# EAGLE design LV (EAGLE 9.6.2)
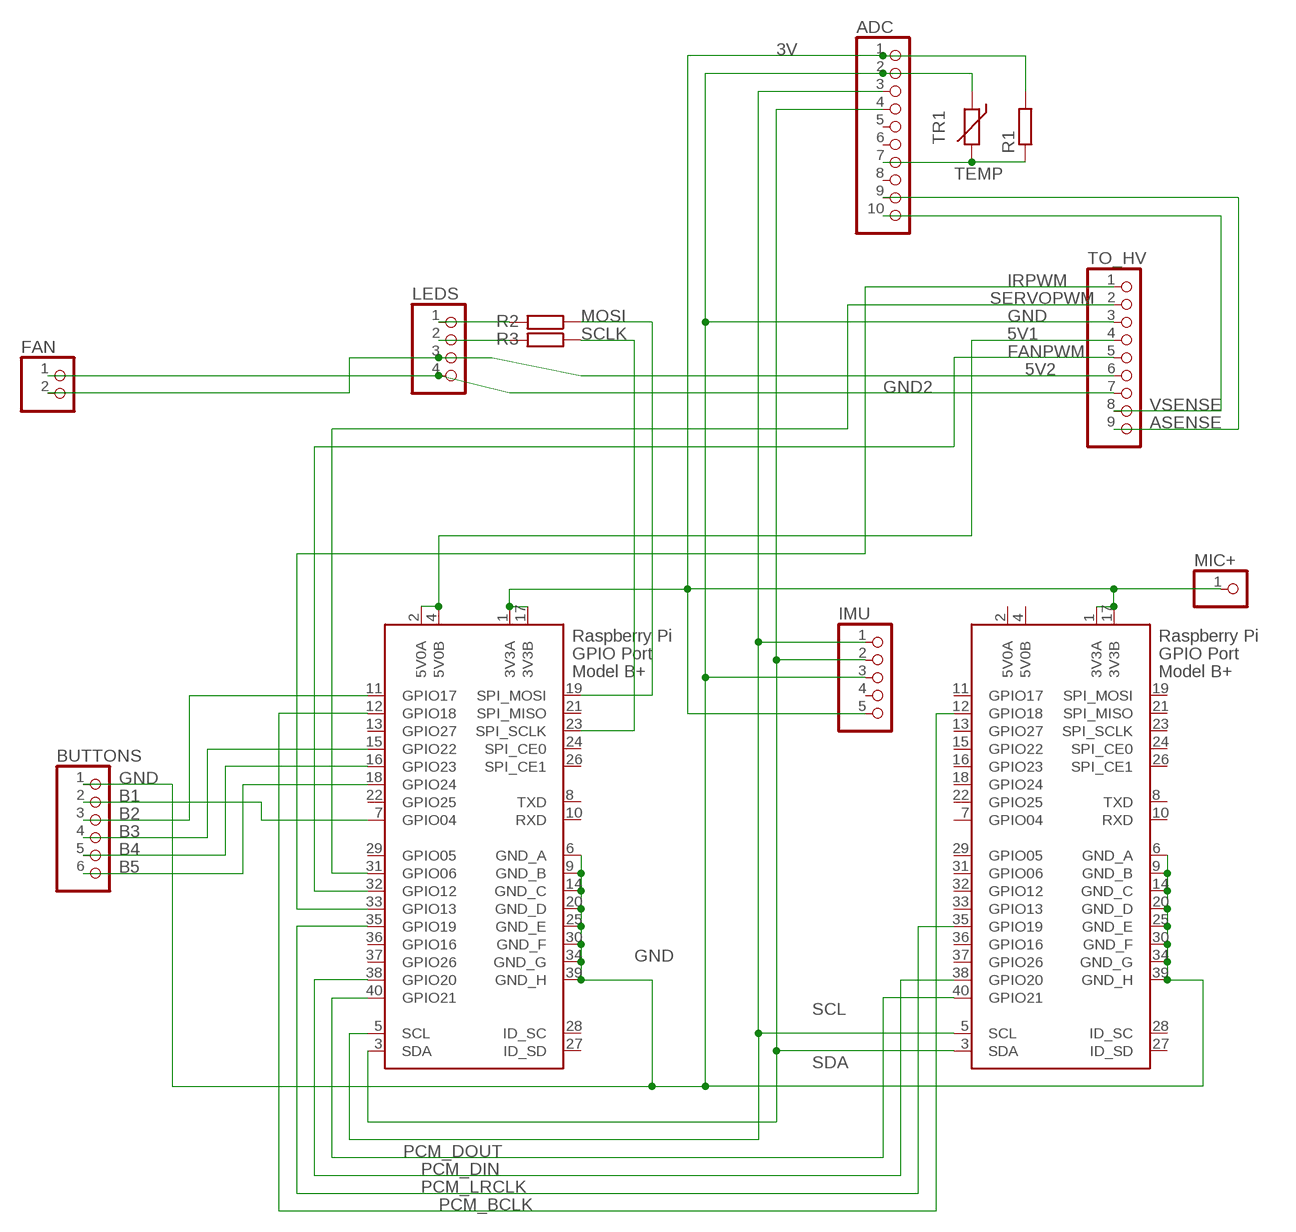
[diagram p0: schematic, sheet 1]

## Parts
ADC  PINHD-1X10  [1X10]
BUTTONS  PINHD-1X6  [1X06]
FAN  PINHD-1X2  [1X02]
IMU  PINHD-1X5  [1X05]
LEDS  PINHD-1X4  [1X04]
MIC+  PINHD-1X1  [1X01]
R1  R-EU_0204/7  [0204/7]
R2  R-EU_0204/7  [0204/7]
R3  R-EU_0204/7  [0204/7]
TO_HV  PINHD-1X9  [1X09]
TR1  THERMISTOR_R-2,5  [RS-2,5]
X1  RASPI_BOARD_B+#_E4P  [RASPI_BOARD_B+_EDGES_4DRILL_PAD]
X2  RASPI_BOARD_B+#F  [FE-PI]

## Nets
3V [PWR]: ADC.1 IMU.5 MIC+.1 R1.2 X1.1(3V3A) X1.17(3V3B) X2.1(3V3A) X2.17(3V3B)
5V1 [PWR]: TO_HV.4 X1.2(5V0A) X1.4(5V0B)
5V2 [PWR]: FAN.2 LEDS.3 TO_HV.6
ASENSE: ADC.9 TO_HV.9
B1: BUTTONS.2 X1.7(GPIO04)
B2: BUTTONS.3 X1.11(GPIO17)
B3: BUTTONS.4 X1.15(GPIO22)
B4: BUTTONS.5 X1.16(GPIO23)
B5: BUTTONS.6 X1.18(GPIO24)
FANPWM: TO_HV.5 X1.32(GPIO12)
GND [PWR]: ADC.2 BUTTONS.1 IMU.3 TO_HV.3 TR1.1 X1.6(GND_A) X1.9(GND_B) X1.14(GND_C) X1.20(GND_D) X1.25(GND_E) X1.30(GND_F) X1.34(GND_G) X1.39(GND_H) X2.6(GND_A) X2.9(GND_B) X2.14(GND_C) X2.20(GND_D) X2.25(GND_E) X2.30(GND_F) X2.34(GND_G) X2.39(GND_H)
GND2 [PWR]: FAN.1 LEDS.4 TO_HV.7
IRPWM: TO_HV.1 X1.33(GPIO13)
MOSI: R2.1 X1.19(SPI_MOSI)
N$6: LEDS.2 R3.2
N$7: LEDS.1 R2.2
PCM_BCLK: X1.12(GPIO18) X2.12(GPIO18)
PCM_DIN: X1.38(GPIO20) X2.38(GPIO20)
PCM_DOUT: X1.40(GPIO21) X2.40(GPIO21)
PCM_LRCLK: X1.35(GPIO19) X2.35(GPIO19)
SCL: ADC.3 IMU.1 X1.5(SCL) X2.5(SCL)
SCLK: R3.1 X1.23(SPI_SCLK)
SDA: ADC.4 IMU.2 X1.3(SDA) X2.3(SDA)
SERVOPWM: TO_HV.2 X1.31(GPIO06)
TEMP: ADC.7 R1.1 TR1.2
VSENSE: ADC.10 TO_HV.8
Unconnected: ADC.5 ADC.6 ADC.8 IMU.4 X1.8(TXD) X1.10(RXD) X1.13(GPIO27) X1.21(SPI_MISO) X1.22(GPIO25) X1.24(SPI_CE0) X1.26(SPI_CE1) X1.27(ID_SD) X1.28(ID_SC) X1.29(GPIO05) X1.36(GPIO16) X1.37(GPIO26) X2.7(GPIO04) X2.8(TXD) X2.10(RXD) X2.11(GPIO17) X2.13(GPIO27) X2.15(GPIO22) X2.16(GPIO23) X2.18(GPIO24) X2.19(SPI_MOSI) X2.21(SPI_MISO) X2.22(GPIO25) X2.23(SPI_SCLK) X2.24(SPI_CE0) X2.26(SPI_CE1) X2.27(ID_SD) X2.28(ID_SC) X2.29(GPIO05) X2.31(GPIO06) X2.32(GPIO12) X2.33(GPIO13) X2.36(GPIO16) X2.37(GPIO26)

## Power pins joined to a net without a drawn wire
5V0A: X2.2(5V0A)
5V0B: X2.4(5V0B)

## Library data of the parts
ADC = pinhead:PINHD-1X10: PIN HEADER
BUTTONS = pinhead:PINHD-1X6: PIN HEADER
FAN = pinhead:PINHD-1X2: PIN HEADER
IMU = pinhead:PINHD-1X5: PIN HEADER
LEDS = pinhead:PINHD-1X4: PIN HEADER
MIC+ = pinhead:PINHD-1X1: PIN HEADER
R1-R3 = rcl:R-EU_: RESISTOR, European symbol; SPICEPREFIX: R
TO_HV = pinhead:PINHD-1X9: PIN HEADER
TR1 = discrete:THERMISTOR_: Thermo Resistor
X1 X2 = raspberrypi_bastelstube_v13:RASPI_BOARD_B+#: Raspberry Pi GPIO connector with markings for the outer dimensions of the Raspberry Pi board model B+ with different sets of drill holes or mounting pads All pins connected

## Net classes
0 default: width 0.152 mm, drill 0.3 mm, clearance 0.178 mm
1 PWR: width 0.381 mm, drill 0.3 mm, clearance 0.152 mm

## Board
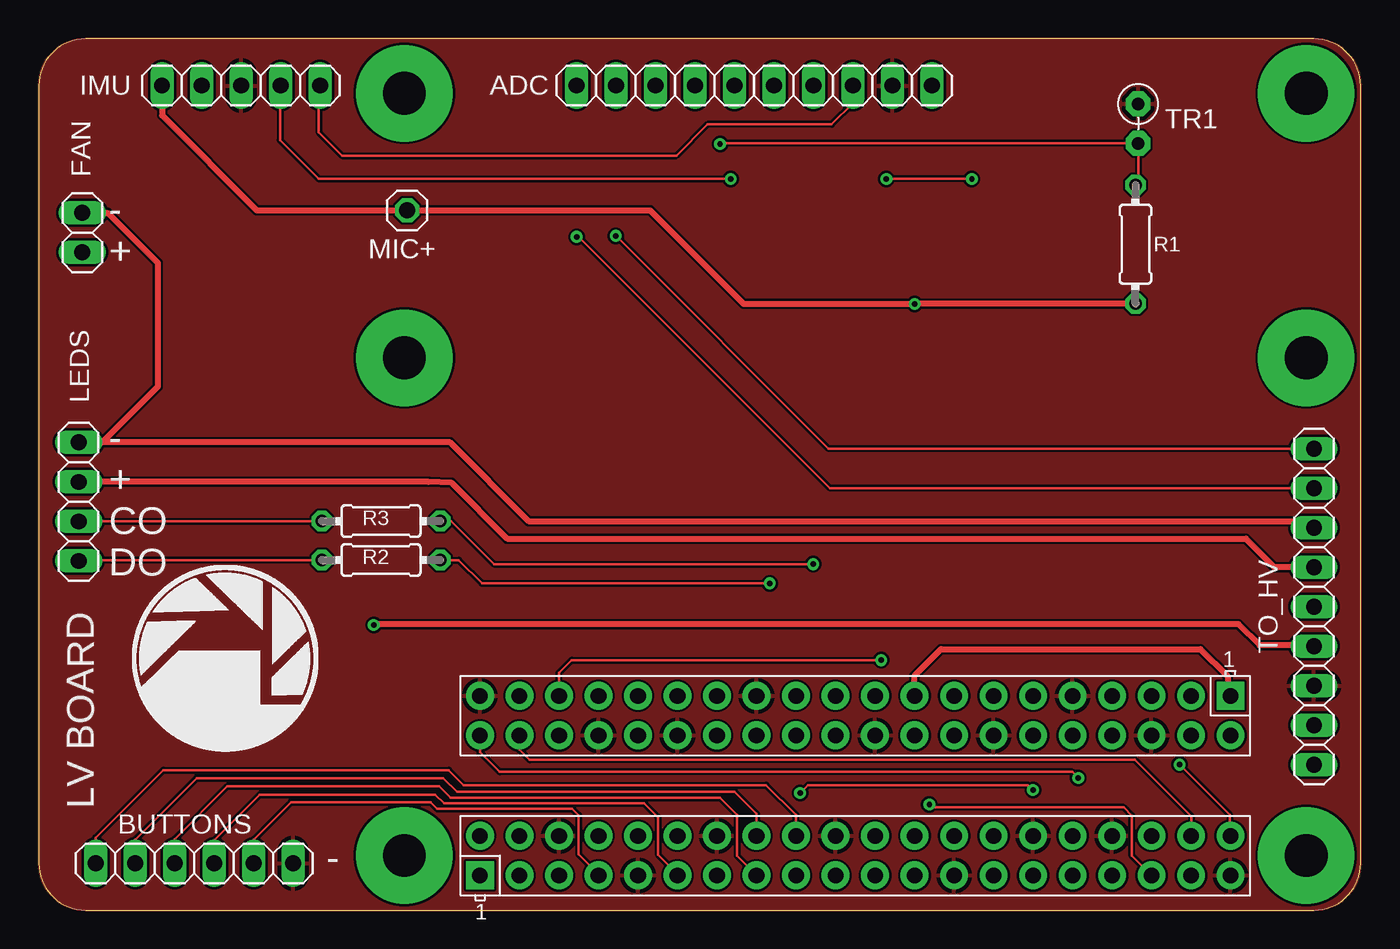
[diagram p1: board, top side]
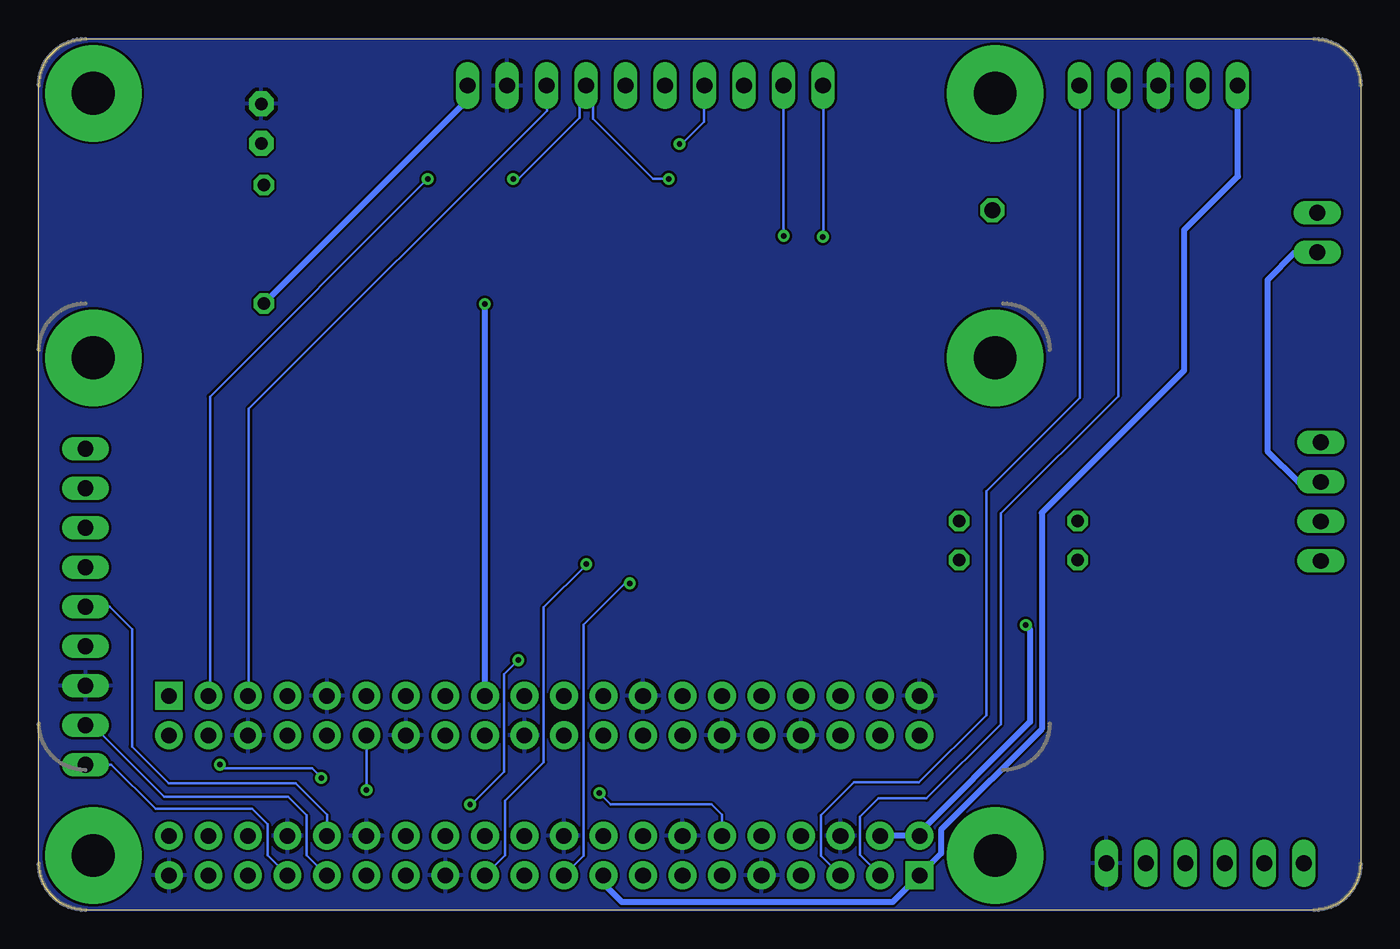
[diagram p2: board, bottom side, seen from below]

Size 85 x 56 mm. Coordinates in mm from the lower left corner, seen from the top.
Outline: 85,3 85,53 arc90 82,56 3,56 arc90 0,53 0,3 arc90 3,0 82,0 arc90 85,3
Copper layers (1*16): Top 0.035mm / dielectric 1.5mm / Bottom 0.035mm
Design rules "default *": minimum track width 6mil, minimum drill 0.35mm, track to track 6mil, track to pad 6mil, pad to pad 6mil, via to via 6mil, smd to smd 6mil, copper to edge 0mil, drill to drill 0.5mm, minimum pad ring 10mil, minimum via ring 8mil, stop-mask expansion 4mil, vias tented up to drill 15mil, thermal gap 10mil

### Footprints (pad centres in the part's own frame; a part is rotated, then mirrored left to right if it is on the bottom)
1X10 = drill 1.016 long: 1 -11.43,0; 2 -8.89,0; 3 -6.35,0; 4 -3.81,0; 5 -1.27,0; 6 1.27,0; 7 3.81,0; 8 6.35,0; 9 8.89,0; 10 11.43,0
1X06 = drill 1.016 long: 1 -6.35,0; 2 -3.81,0; 3 -1.27,0; 4 1.27,0; 5 3.81,0; 6 6.35,0
1X02 = drill 1.016 long: 1 -1.27,0; 2 1.27,0
1X05 = drill 1.016 long: 1 -5.08,0; 2 -2.54,0; 3 0,0; 4 2.54,0; 5 5.08,0
1X04 = drill 1.016 long: 1 -3.81,0; 2 -1.27,0; 3 1.27,0; 4 3.81,0
1X01 = drill 1.016 octagon: 1 0,0
0204/7 = drill 0.813 octagon: 1 -3.81,0; 2 3.81,0
1X09 = drill 1.016 long: 1 -10.16,0; 2 -7.62,0; 3 -5.08,0; 4 -2.54,0; 5 0,0; 6 2.54,0; 7 5.08,0; 8 7.62,0; 9 10.16,0
RS-2,5 = drill 0.813 pad 1.6 octagon: 1 -1.27,0; 2 1.27,0
RASPI_BOARD_B+_EDGES_4DRILL_PAD = drill 1 pad 1.778 square: 1 56.63,53.77 | drill 1 pad 1.778: 2 56.63,51.23; 3 54.09,53.77; 4 54.09,51.23; 5 51.55,53.77; 6 51.55,51.23; 7 49.01,53.77; 8 49.01,51.23; 9 46.47,53.77; 10 46.47,51.23; 11 43.93,53.77; 12 43.93,51.23; 13 41.39,53.77; 14 41.39,51.23; 15 38.85,53.77; 16 38.85,51.23; 17 36.31,53.77; 18 36.31,51.23; 19 33.77,53.77; 20 33.77,51.23; 21 31.23,53.77; 22 31.23,51.23; 23 28.69,53.77; 24 28.69,51.23; 25 26.15,53.77; 26 26.15,51.23; 27 23.61,53.77; 28 23.61,51.23; 29 21.07,53.77; 30 21.07,51.23; 31 18.53,53.77; 32 18.53,51.23; 33 15.99,53.77; 34 15.99,51.23; 35 13.45,53.77; 36 13.45,51.23; 37 10.91,53.77; 38 10.91,51.23; 39 8.37,53.77; 40 8.37,51.23 | drill 2.75 pad 6.2: 41 3.5,3.5; 42 61.5,3.5; 43 61.5,52.5; 44 3.5,52.5
FE-PI = drill 1 pad 1.778 square: 1 8.37,25.23 | drill 1 pad 1.778: 2 8.37,27.77; 3 10.91,25.23; 4 10.91,27.77; 5 13.45,25.23; 6 13.45,27.77; 7 15.99,25.23; 8 15.99,27.77; 9 18.53,25.23; 10 18.53,27.77; 11 21.07,25.23; 12 21.07,27.77; 13 23.61,25.23; 14 23.61,27.77; 15 26.15,25.23; 16 26.15,27.77; 17 28.69,25.23; 18 28.69,27.77; 19 31.23,25.23; 20 31.23,27.77; 21 33.77,25.23; 22 33.77,27.77; 23 36.31,25.23; 24 36.31,27.77; 25 38.85,25.23; 26 38.85,27.77; 27 41.39,25.23; 28 41.39,27.77; 29 43.93,25.23; 30 43.93,27.77; 31 46.47,25.23; 32 46.47,27.77; 33 49.01,25.23; 34 49.01,27.77; 35 51.55,25.23; 36 51.55,27.77; 37 54.09,25.23; 38 54.09,27.77; 39 56.63,25.23; 40 56.63,27.77 | drill 2.75 pad 6.2: 41 3.5,3.5; 42 61.5,3.5

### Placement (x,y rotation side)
ADC  46,53 180 top
BUTTONS  10,3 180 top
FAN  2.79,43.55 270 top
IMU  13,53 180 top
LEDS  2.56,26.25 90 top
MIC+  23.68,44.98 180 top
R1  70.52,42.8 270 top
R2  22,22.5 180 top
R3  22,25 180 top
TO_HV  82,19.5 90 top
TR1  70.69,50.55 270 top
X1  85,56 180 top
X2  85,39 180 top

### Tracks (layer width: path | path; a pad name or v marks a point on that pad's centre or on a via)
3V  (via drill 0.35)
  Top 0.381: X2.1 76.45,13.95 76.45,15.02 74.69,16.77 58.01,16.77 56.31,15.07 X2.17 | R1.2 70.49,38.96 v56.33,38.96 45.33,38.96 39.31,44.98 MIC+.1 14.02,44.98 7.92,51.08 IMU.5
  Bottom 0.381: X2.17 56.31,38.94 v56.33,38.96 | R1.2 57.43,52.08 ADC.1 | IMU.5 7.9,53.01 7.9,47.17 11.34,43.73 11.34,34.7 20.5,25.54 20.5,11.63 26.99,5.14 26.99,3.63 28.37,2.25 X1.1 30.1,0.5 47.5,0.5 48.69,1.69 X1.17
5V1  (via drill 0.35)
  Top 0.381: v21.53,18.32 21.59,18.38 77.14,18.38 78.51,17.02 81.94,17.02 TO_HV.4
  Bottom 0.381: v21.53,18.32 21.25,18.05 21.25,12.09 28.54,4.81 28.41,4.81 X1.2 X1.4
5V2
  Top 0.381: TO_HV.6 79.46,22.04 77.62,23.88 30.12,23.88 26.55,27.45 25.06,27.52 LEDS.3
  Bottom 0.381: LEDS.3 4.02,27.52 6,29.5 6,40.5 4.22,42.28 FAN.2
ASENSE  (via drill 0.35)
  Top 0.152: v37.1,43.34 50.78,29.66 TO_HV.9
  Bottom 0.152: ADC.9 v37.1,43.34
B1
  Top 0.152: BUTTONS.2 13.81,4.52 16.22,6.93 25.18,6.93 25.61,6.5 34.3,6.5 34.7,6.09 34.7,3.57 35.99,2.29 X1.7
B2
  Top 0.152: BUTTONS.3 11.27,4.47 14.21,7.42 25.49,7.42 26.04,6.86 38.92,6.86 39.82,5.96 39.82,3.55 41.07,2.3 X1.11
B3
  Top 0.152: BUTTONS.4 8.73,4.55 12.12,7.95 25.74,7.95 26.47,7.22 43.81,7.22 44.9,6.14 44.9,3.48 X1.15
B4
  Top 0.152: BUTTONS.5 6.19,4.53 10.14,8.48 26,8.48 26.88,7.6 44.72,7.6 46.15,6.17 X1.16
B5
  Top 0.152: BUTTONS.6 3.65,4.65 8,9 26.35,9 27.32,8.03 46.77,8.03 48.69,6.12 X1.18
FANPWM
  Bottom 0.152: TO_HV.5 80.44,19.5 79,18.06 79,10.5 76.64,8.14 68.48,8.14 66.47,6.13 X1.32
GND
  pour Bottom: 0,3 0,53 arc-90 3,56 82,56 arc-90 85,53 85,3 arc-90 82,0 3,0 arc-90
  pour Top: 85,53 85,3 arc-90 82,0 3,0 arc-90 0,3 0,53 arc-90 3,56 82,56 arc-90
GND2
  Top 0.381: FAN.1 4.42,44.82 7.64,41.59 7.64,33.64 4.06,30.06 LEDS.4 26.44,30.06 31.5,25 82,25 TO_HV.7
IRPWM
  Bottom 0.152: X1.33 70.29,3.51 70.29,5.52 71.27,6.5 77.5,6.5 80.34,9.34 TO_HV.1
MOSI  (via drill 0.35)
  Top 0.152: v47,21 28.5,21 27,22.5 R2.1
  Bottom 0.152: v47,21 47.31,21 49.96,18.35 49.96,3.5 X1.19
N$6
  Top 0.152: LEDS.2 2.58,25 R3.2
N$7
  Top 0.152: R2.2 2.62,22.5 LEDS.1
PCM_BCLK  (via drill 0.35)
  Top 0.152: v48.95,7.52 49.46,8.03 63.61,8.03 v63.93,7.71
  Bottom 0.152: v48.95,7.52 48.23,6.8 41.75,6.8 41.07,6.12 X1.12 | X2.12 | X2.12 v63.93,7.71
PCM_DIN
  Top 0.152: X1.38 74.1,4.78 74.1,6.04 70.49,9.65 31.56,9.65 30.91,10.3 X2.38
PCM_DOUT  (via drill 0.35 pad 0.6)
  Top 0.152: X1.40 76.58,4.77 76.58,6.13 v73.36,9.35 | X2.40 28.37,10.13 29.63,8.87 66.45,8.87 v66.84,8.49 v66.84,8.48
  Bottom 0.152: v73.36,9.35 73.12,9.1 67.43,9.1 67.07,8.74 67.07,8.71 v66.84,8.48
PCM_LRCLK  (via drill 0.35)
  Top 0.152: X1.35 70.29,3.49 70.29,6.07 69.76,6.59 57.46,6.59 v57.27,6.78 | X2.35 33.45,15.25 34.27,16.06 v54.17,16.06
  Bottom 0.152: v57.27,6.78 57.16,6.78 55.07,8.88 55.07,15.16 v54.17,16.06
SCL
  Top 0.152: IMU.1 18,52.92 18,50 19.5,48.5 41,48.5 43,50.5 50.98,50.5 52.35,51.87 ADC.3
  Bottom 0.152: ADC.3 52.33,52.98 52.33,51.4 71.5,32.23 71.5,14 X2.5 | IMU.1 18.06,52.98 18.06,32.94 24.07,26.93 24.07,12.53 28.39,8.21 32.59,8.21 34.71,6.1 34.71,3.49 X1.5
SCLK  (via drill 0.35)
  Top 0.152: v49.79,22.23 29.27,22.23 26.5,25 R3.1
  Bottom 0.152: v49.79,22.23 49.79,22.21 52.53,19.47 52.53,9.51 55.02,7.01 55.02,3.52 X1.23
SDA  (via drill 0.35)
  Top 0.152: IMU.2 15.5,52.96 15.5,49.5 18,47 v44.5,47 | v60,47 v54.5,47
  Bottom 0.152: v44.5,47 45.5,47 49.37,50.87 49.37,52.56 ADC.4 50.23,52.59 50.23,50.94 54.17,47 v54.5,47 | v60,47 74,33 74,14 X2.3 | X1.3 30.91,2.3 30.91,2.27 32.19,3.55 32.19,6 31.02,7.17 27.91,7.17 23.14,11.95 23.14,25.49 15.59,33.04 15.59,52.95 IMU.2
SERVOPWM
  Bottom 0.152: TO_HV.2 81.97,11.9 81.57,11.9 76.94,7.28 68.98,7.28 67.78,6.08 67.78,3.51 66.5,2.23 X1.31
TEMP  (via drill 0.35)
  Top 0.152: R1.1 70.69,46.78 TR1.2 43.84,49.28 v43.8,49.24
  Bottom 0.152: v43.8,49.24 43.73,49.17 42.22,50.67 42.22,53 ADC.7
VSENSE  (via drill 0.35)
  Top 0.152: v34.58,43.28 34.65,43.35 50.88,27.12 51.88,27.12 TO_HV.8
  Bottom 0.152: ADC.10 34.54,52.97 34.54,43.32 v34.58,43.28

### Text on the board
tNames: - / + | - / + / CO / DO | LV BOARD | -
